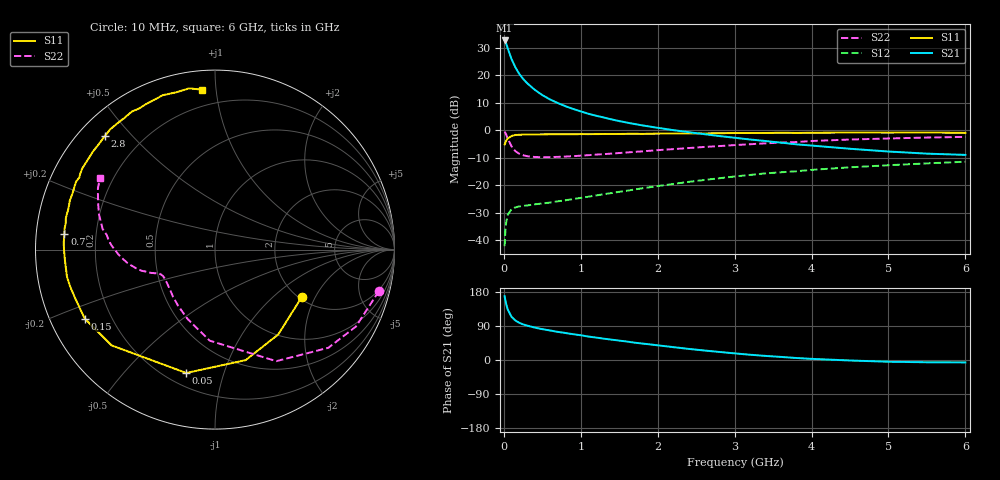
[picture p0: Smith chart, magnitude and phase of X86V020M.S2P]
! SIEMENS Small Signal Semiconductors
! BFP136W
! Si NPN RF Bipolar Junction Transistor in SOT343
! VCE = 6 V  IC = 20 mA
! Common Emitter S-Parameters:  September  1994
# GHz  S  MA  R  50
!  f  S11  S21  S12  S22
! GHz  MAG  ANG  MAG  ANG  MAG  ANG  MAG  ANG
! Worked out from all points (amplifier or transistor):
!   40 points, 10 MHz to 6 GHz, reference 50 ohm
!   highest |S21| = 32.6 dB at 10 MHz (marker M1)
!   |S21| within 3 dB of that: start of sweep to 52.4 MHz
!   unconditionally stable (mu >= 1): 881 MHz to 2.781 GHz
!   at 200 MHz: K = 0.32, MSG = 24.1 dB, |S12| = -27.7 dB
!   at 1.5 GHz: K = 1.16, MAG = 10.4 dB, |S12| = -22.4 dB
!   at 6 GHz: K = 0.97, MSG = 1.2 dB, |S12| = -11.5 dB
!   S11 on the Smith chart (normalised r, x): 10 MHz: 2.07, -1.57; 50 MHz: 0.28, -0.76; 150 MHz: 0.10, -0.25; 700 MHz: 0.08, +0.05; 2.8 GHz: 0.07, +0.42; 6 GHz: 0.10, +0.92
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0.01  0.551 -28.7  42.81 168.6  0.0078 78.0  0.9421 -14.2
0.02  0.5897 -53.3  40.07 157.7  0.0149 68.9  0.8948 -28.6
0.03  0.639 -74.5  37.58 148.4  0.0209 60.2  0.8355 -40.9
0.05  0.7057 -103.1  30.98 133.6  0.0288 47.1  0.7093 -61.2
0.1  0.7855 -137.2  19.64 113.9  0.037 32.1  0.5083 -93.3
0.15  0.8211 -152.1  13.89 104.2  0.0395 27.0  0.4156 -111.6
0.2  0.8243 -160.3  10.59 98.2  0.0413 24.7  0.3734 -123.6
0.25  0.8331 -165.8  8.596 94.0  0.042 24.3  0.3514 -131.8
0.3  0.8384 -169.5  7.217 90.9  0.0428 24.8  0.3371 -137.6
0.4  0.8381 -175.5  5.447 85.6  0.0449 26.6  0.3262 -145.1
0.5  0.8409 -179.6  4.352 81.4  0.0466 28.5  0.3231 -149.7
0.6  0.8437 177.5  3.629 77.9  0.0484 31.0  0.3243 -152.4
0.7  0.8437 174.2  3.125 74.3  0.051 34.1  0.3277 -154.2
0.9  0.8447 170.0  2.438 68.1  0.056 38.1  0.3373 -156.7
1.1  0.8479 165.1  1.989 61.8  0.0619 42.0  0.3518 -158.0
1.6  0.8587 155.7  1.375 48.7  0.0794 48.6  0.3941 -161.4
2.2  0.8677 145.1  1.005 34.0  0.1053 51.1  0.4527 -166.8
2.8  0.8816 134.1  0.784 21.3  0.1339 49.8  0.5146 -174.1
3.2  0.8892 127.5  0.678 13.9  0.1536 47.2  0.5559 -179.6
4.5  0.9079 108.7  0.46 -1.3  0.2116 36.7  0.6769 162.9
5.5  0.9097 99.1  0.375 -6.0  0.2497 28.1  0.7361 152.4
6  0.8941 94.6  0.356 -6.4  0.2676 23.5  0.7555 148.0
